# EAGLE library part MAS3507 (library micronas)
MPEG3 DECODER
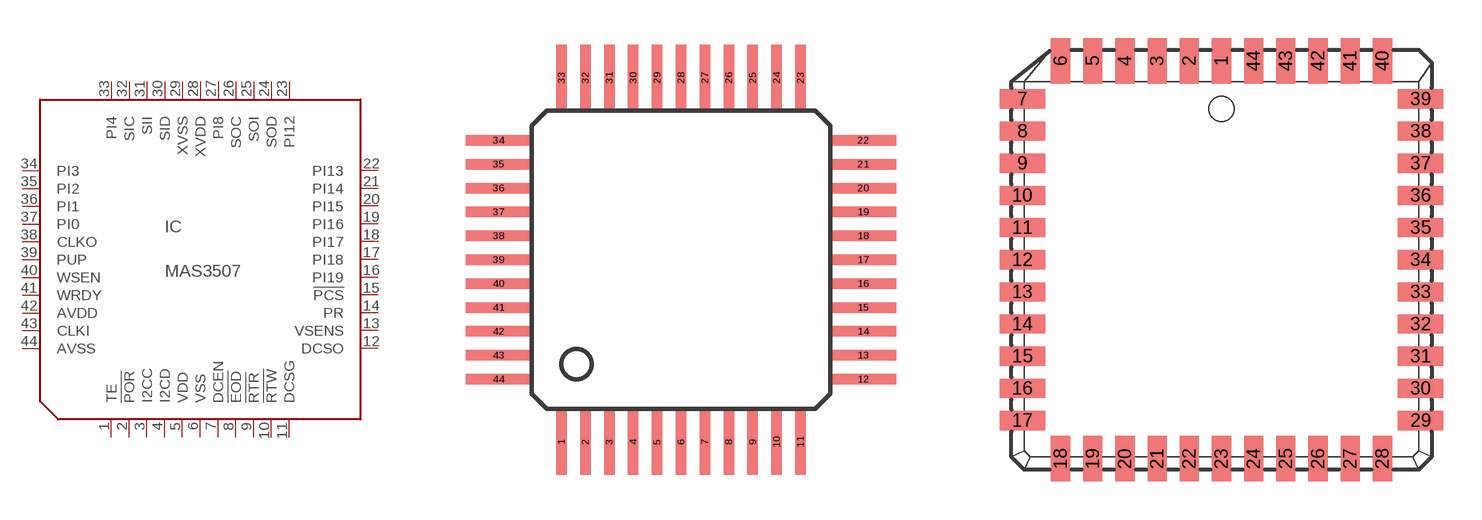
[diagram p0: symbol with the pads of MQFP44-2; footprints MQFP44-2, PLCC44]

Designator prefix IC

## MAS3507D (OC_FARNELL: unknown; OC_NEWARK: unknown)  [MQFP44-2]
1  TE  in
2  !POR  in
3  I2CC
4  I2CD
5  VDD  pwr
6  VSS  pwr
7  DCEN  in
8  !EOD  out
9  !RTR  out
10  !RTW  out
11  DCSG  pwr
12  DCSO  out
13  VSENS  in
14  PR  in
15  !PCS  in
16  PI19
17  PI18
18  PI17
19  PI16
20  PI15
21  PI14
22  PI13
23  PI12
24  SOD  out
25  SOI  out
26  SOC  out
27  PI8
28  XVDD  pwr
29  XVSS  pwr
30  SID  in
31  SII  in
32  SIC  in
33  PI4
34  PI3
35  PI2
36  PI1
37  PI0
38  CLKO  out
39  PUP  out
40  WSEN  in
41  WRDY  out
42  AVDD  pwr
43  CLKI  in
44  AVSS  pwr

## MAS3507J (OC_FARNELL: unknown; OC_NEWARK: unknown)  [PLCC44]
1  VSS  pwr
2  VDD  pwr
3  I2CD
4  I2CC
5  !POR  in
6  TE  in
7  AVSS  pwr
8  CLKI  in
9  AVDD  pwr
10  WRDY  out
11  WSEN  in
12  PUP  out
13  CLKO  out
14  PI0
15  PI1
16  PI2
17  PI3
18  PI4
19  SIC  in
20  SII  in
21  SID  in
22  XVSS  pwr
23  XVDD  pwr
24  PI8
25  SOC  out
26  SOI  out
27  SOD  out
28  PI12
29  PI13
30  PI14
31  PI15
32  PI16
33  PI17
34  PI18
35  PI19
36  !PCS  in
37  PR  in
38  VSENS  in
39  DCSO  out
40  DCSG  pwr
41  !RTW  out
42  !RTR  out
43  !EOD  out
44  DCEN  in

## Footprint MQFP44-2 (pad centres in mm)
Metric Quad Flat Pack
smd 0.35 x 2.2: 1 -4,-6.1; 2 -3.2,-6.1; 3 -2.4,-6.1; 4 -1.6,-6.1; 5 -0.8,-6.1; 6 0,-6.1; 7 0.8,-6.1; 8 1.6,-6.1; 9 2.4,-6.1; 10 3.2,-6.1; 11 4,-6.1; 23 4,6.1; 24 3.2,6.1; 25 2.4,6.1; 26 1.6,6.1; 27 0.8,6.1; 28 0,6.1; 29 -0.8,6.1; 30 -1.6,6.1; 31 -2.4,6.1; 32 -3.2,6.1; 33 -4,6.1
smd 2.2 x 0.35: 12 6.1,-4; 13 6.1,-3.2; 14 6.1,-2.4; 15 6.1,-1.6; 16 6.1,-0.8; 17 6.1,0; 18 6.1,0.8; 19 6.1,1.6; 20 6.1,2.4; 21 6.1,3.2; 22 6.1,4; 34 -6.1,4; 35 -6.1,3.2; 36 -6.1,2.4; 37 -6.1,1.6; 38 -6.1,0.8; 39 -6.1,0; 40 -6.1,-0.8; 41 -6.1,-1.6; 42 -6.1,-2.4; 43 -6.1,-3.2; 44 -6.1,-4

## Footprint PLCC44 (pad centres in mm)
PLASTIC LEADED CHIP CARRIER square
smd 0.76 x 1.8: 1 0,7.86; 2 -1.27,7.86; 3 -2.54,7.86; 4 -3.81,7.86; 5 -5.08,7.86; 6 -6.35,7.86; 18 -6.35,-7.86; 19 -5.08,-7.86; 20 -3.81,-7.86; 21 -2.54,-7.86; 22 -1.27,-7.86; 23 0,-7.86; 24 1.27,-7.86; 25 2.54,-7.86; 26 3.81,-7.86; 27 5.08,-7.86; 28 6.35,-7.86; 40 6.35,7.86; 41 5.08,7.86; 42 3.81,7.86; 43 2.54,7.86; 44 1.27,7.86
smd 1.8 x 0.76: 7 -7.86,6.35; 8 -7.86,5.08; 9 -7.86,3.81; 10 -7.86,2.54; 11 -7.86,1.27; 12 -7.86,0; 13 -7.86,-1.27; 14 -7.86,-2.54; 15 -7.86,-3.81; 16 -7.86,-5.08; 17 -7.86,-6.35; 29 7.86,-6.35; 30 7.86,-5.08; 31 7.86,-3.81; 32 7.86,-2.54; 33 7.86,-1.27; 34 7.86,0; 35 7.86,1.27; 36 7.86,2.54; 37 7.86,3.81; 38 7.86,5.08; 39 7.86,6.35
